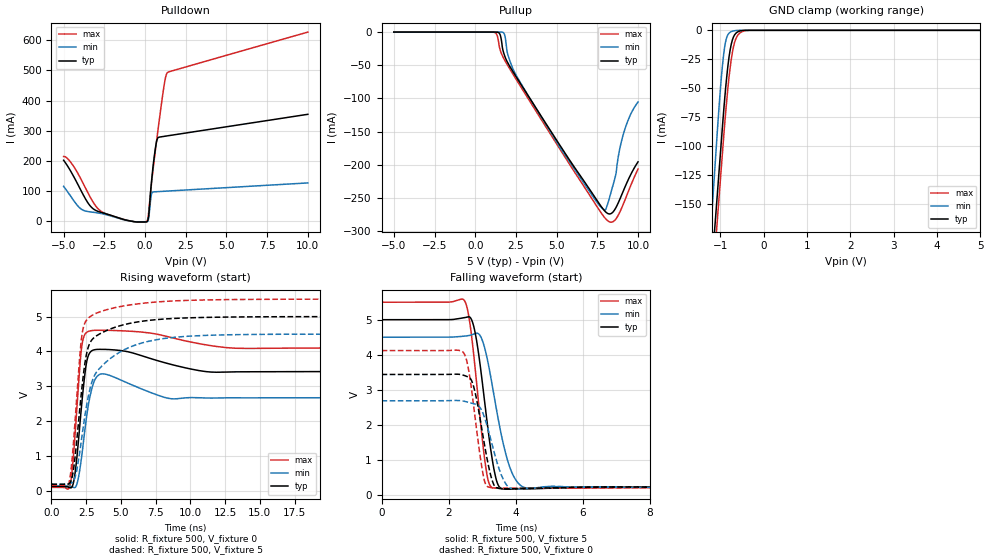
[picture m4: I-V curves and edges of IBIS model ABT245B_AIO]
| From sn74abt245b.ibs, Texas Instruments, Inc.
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[Model]   ABT245B_AIO
Model_type  I/O
Vinl=0.8
Vinh=2.0
Enable   Active-Low
Vref =   0
Rref =   500
Cref =   50p
Vmeas =   1.5
| variable   typ   min   max
C_comp   5.08pF   3.90pF   7.83pF
| C_pullup   5.58pF   4.35pF   8.31pF
| C_pulldown   8.93pF   0.50pF   29.81pF
| C_tri-state   5.08pF   3.90pF   7.83pF
[Temperature Range]   40   -40   100
| Ambient temperature   25   -40   85
[Voltage range]   5   4.5   5.5
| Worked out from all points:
|   slope of the pulldown table from 0 to 0.75 V, typ, clamps not added: 2.73 ohm
|   GND clamp passes 1 mA (typ) near -0.58 V on its own axis
|   rising waveform, R_fixture 500, V_fixture 0: 20-80 % time 461ps typ, 487ps min, 434ps max; typ from 0.141 V to 3.43 V
|   falling waveform, R_fixture 500, V_fixture 5: 20-80 % time 384ps typ, 528ps min, 348ps max; typ from 5 V to 0.203 V
|   rising waveform, R_fixture 500, V_fixture 5: 20-80 % time 843ps typ, 1.76ns min, 628ps max; typ from 0.201 V to 5 V
|   falling waveform, R_fixture 500, V_fixture 0: 20-80 % time 367ps typ, 450ps min, 325ps max; typ from 3.43 V to 0.179 V
[GND Clamp]
| ABT245B_AIO
|   Voltage   I(typ)   I(min)   I(max)
-5V       -2.316A    -2.434A    -2.364A
-1.33V    -270.9mA   -233.6mA   -293.2mA
-1.2V     -205.8mA   -159.9mA   -228.2mA
-1.135V   -173.4mA   -123.1mA   -195.8mA
-1.075V   -143.6mA   -89.24mA   -166.1mA
-1V       -106.4mA   -50.47mA   -129mA
-925mV    -69.65mA   -20.53mA   -92.09mA
-825mV    -29.95mA   -3.59mA    -48.89mA
-750mV    -12.01mA   -1.121mA   -25.21mA
-625mV    -1.924mA   -89.6uA    -5.767mA
-400mV    -6.785uA   -3.043nA   -156.2uA
5V        82.37pA    74.89pA    1.482nA
[Pulldown]
| ABT245B_AIO
|   Voltage   I(typ)   I(min)   I(max)
-5V       202.3mA    115.6mA    214.8mA
-3.995V   108.4mA    43.59mA    145.9mA
-3.175V   40.93mA    29.77mA    62.18mA
-2.36V    24.13mA    21.39mA    24mA
80mV      -1.968mA   -1.512mA   -2.066mA
215mV     14.81mA    8.02mA     25.44mA
415mV     141.1mA    93.33mA    134.1mA
570mV     216.1mA    97.56mA    206.9mA
720mV     266.7mA    98.04mA    271mA
1.165V    281.4mA    99.43mA    448.1mA
1.365V    283.1mA    100.1mA    492.2mA
10V       354.6mA    127.1mA    627.2mA
[Pullup]
| ABT245B_AIO
|   Voltage   I(typ)   I(min)   I(max)
-5V       -3.55pA    -3.231pA   -5.44pA
1.17V     -6.217uA   -450pA     -388.2uA
1.35V     -173.1uA   -69.35nA   -5.383mA
1.52V     -3.386mA   -5.427uA   -25.69mA
1.735V    -30.1mA    -916.7uA   -38.91mA
2.035V    -47.84mA   -36.39mA   -51.92mA
2.6V      -70.64mA   -68.73mA   -74.52mA
5.73V     -190.4mA   -193.2mA   -196.6mA
7.955V    -269.5mA   -267.8mA   -279.6mA
8.67V     -263.1mA   -208.8mA   -280.4mA
9.18V     -234.5mA   -147.1mA   -254mA
10V       -195.4mA   -105.3mA   -206.4mA
[Ramp]
| ABT245B_AIO
| variable   typ   min   max
dV/dt_r   2.37/5.72E-10   1.95/6.81E-10   2.73/4.96E-10
dV/dt_f   2.96/3.98E-10   2.66/5.48E-10   3.25/3.57E-10
R_load = 500
[Rising Waveform]
| ABT245B_AIO
R_fixture =   500
C_fixture =   0
L_fixture =   0
V_fixture =   0
V_fixture_min = 0
V_fixture_max = 0
|   Time   V(typ)   V(min)   V(max)
0s        141.4mV    160.3mV    117.2mV
1.34ns    107.5mV    144.7mV    177.4mV
1.69ns    486mV      110.1mV    1.557V
2.165ns   2.428V     961.9mV    4.084V
2.46ns    3.511V     1.92V      4.517V
2.67ns    3.894V     2.493V     4.575V
3.1ns     4.05V      3.168V     4.604V
3.67ns    4.06V      3.361V     4.606V
8.645ns   3.628V     2.648V     4.396V
24.99ns   3.43V      2.679V     4.107V
[Falling Waveform]
| ABT245B_AIO
R_fixture =   500
C_fixture =   0
L_fixture =   0
V_fixture =   5
V_fixture_min = 4.5
V_fixture_max = 5.5
|   Time   V(typ)   V(min)   V(max)
0s        5V         4.5V       5.5V
2.475ns   5.06V      4.531V     5.538V
2.62ns    5.079V     4.552V     4.978V
2.795ns   4.6V       4.604V     3.554V
3.105ns   2.395V     4.072V     794.4mV
3.31ns    942.1mV    3.064V     186.3mV
3.49ns    247.2mV    2.095V     178.2mV
3.805ns   154.2mV    830mV      170.7mV
4.325ns   162.8mV    186.9mV    172.2mV
24.99ns   203.5mV    216.9mV    188.1mV
[Rising Waveform]
| ABT245B_AIO
R_fixture =   500
C_fixture =   0
L_fixture =   0
V_fixture =   5
V_fixture_min = 4.5
V_fixture_max = 5.5
|   Time   V(typ)   V(min)   V(max)
0s        200.8mV    216.8mV    178.7mV
1.28ns    222.9mV    224.8mV    271.1mV
1.62ns    714.1mV    321.2mV    1.561V
2.025ns   2.292V     1.087V     3.771V
2.195ns   2.958V     1.569V     4.462V
2.555ns   3.977V     2.512V     4.91V
3ns       4.371V     3.225V     5.05V
4.93ns    4.736V     3.985V     5.282V
7.965ns   4.923V     4.363V     5.427V
24.99ns   4.999V     4.499V     5.499V
[Falling Waveform]
| ABT245B_AIO
R_fixture =   500
C_fixture =   0
L_fixture =   0
V_fixture =   0
V_fixture_min = 0
V_fixture_max = 0
|   Time   V(typ)   V(min)   V(max)
0s        3.434V     2.681V     4.117V
2.44ns    3.413V     2.672V     4.059V
2.58ns    3.364V     2.639V     3.639V
2.75ns    3.068V     2.596V     2.5V
3.055ns   1.498V     2.241V     439.4mV
3.255ns   544.3mV    1.578V     200.6mV
3.385ns   223.1mV    1.11V      189.2mV
3.61ns    168.6mV    472mV      182.8mV
3.93ns    168.5mV    162mV      179.5mV
24.99ns   179mV      166.6mV    173.6mV
